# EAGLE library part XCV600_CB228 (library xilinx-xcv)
xcv600_cb228 edit this description Auto generated by make-symbol-device-package-bsdl.ulp Rev. 26 Source: xcv600_cb228.bsd
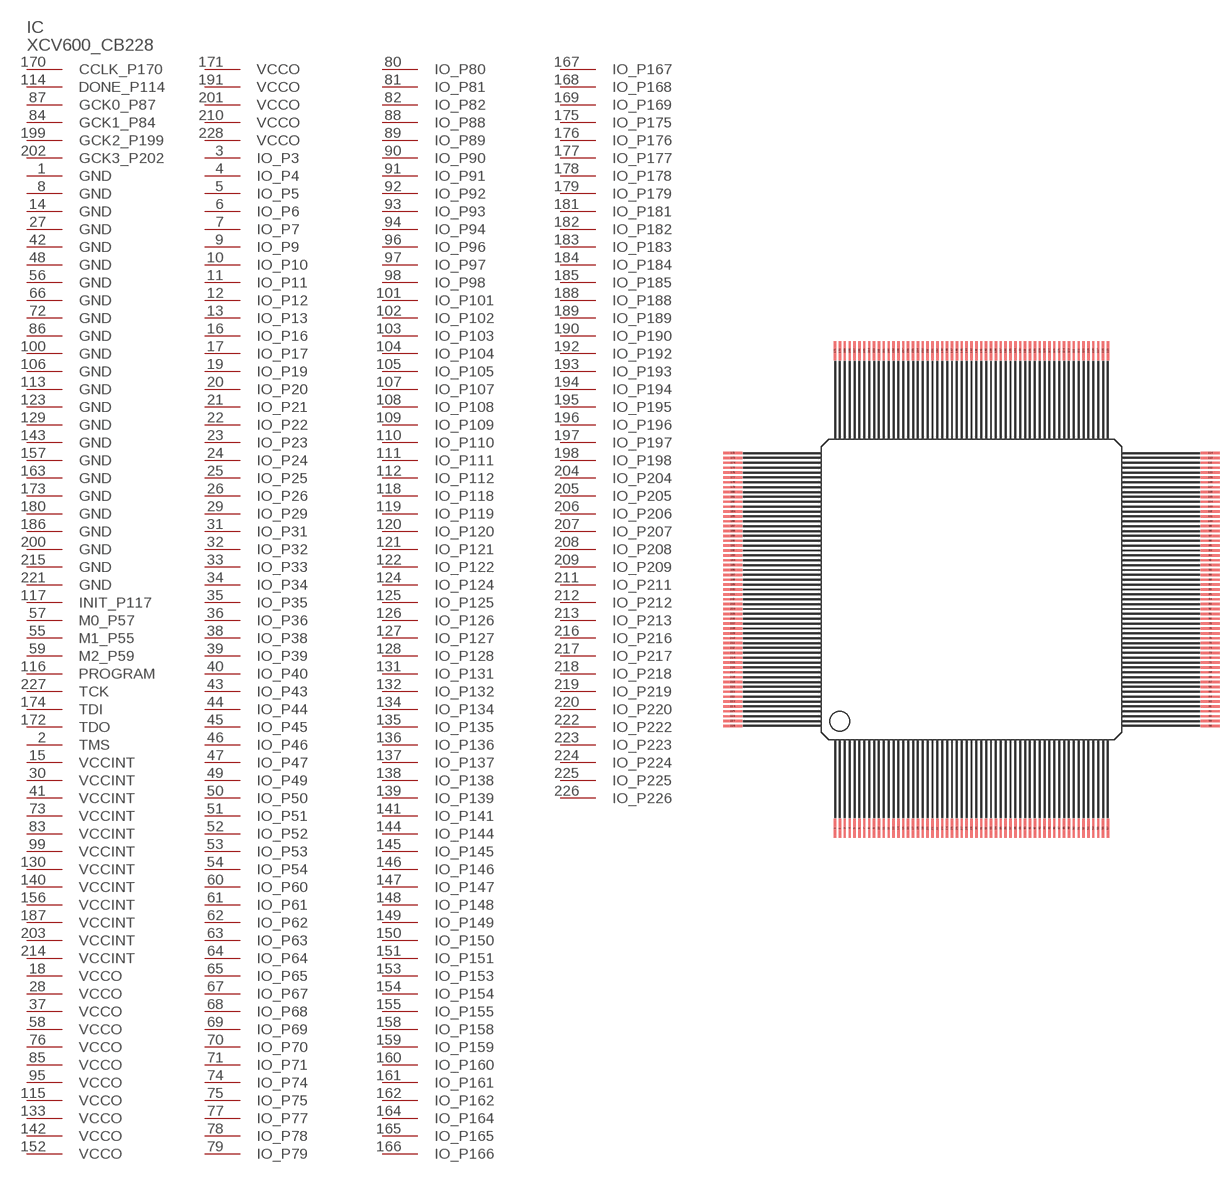
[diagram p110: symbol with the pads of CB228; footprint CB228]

Designator prefix IC

## XCV600_CB228 (OC_FARNELL: unknown; OC_NEWARK: unknown)  [CB228]
1  GND  pwr
2  TMS  in
3  IO_P3
4  IO_P4
5  IO_P5
6  IO_P6
7  IO_P7
8  GND  pwr
9  IO_P9
10  IO_P10
11  IO_P11
12  IO_P12
13  IO_P13
14  GND  pwr
15  VCCINT  pwr
16  IO_P16
17  IO_P17
18  VCCO  pwr
19  IO_P19
20  IO_P20
21  IO_P21
22  IO_P22
23  IO_P23
24  IO_P24
25  IO_P25
26  IO_P26
27  GND  pwr
28  VCCO  pwr
29  IO_P29
30  VCCINT  pwr
31  IO_P31
32  IO_P32
33  IO_P33
34  IO_P34
35  IO_P35
36  IO_P36
37  VCCO  pwr
38  IO_P38
39  IO_P39
40  IO_P40
41  VCCINT  pwr
42  GND  pwr
43  IO_P43
44  IO_P44
45  IO_P45
46  IO_P46
47  IO_P47
48  GND  pwr
49  IO_P49
50  IO_P50
51  IO_P51
52  IO_P52
53  IO_P53
54  IO_P54
55  M1_P55  in
56  GND  pwr
57  M0_P57  in
58  VCCO  pwr
59  M2_P59  in
60  IO_P60
61  IO_P61
62  IO_P62
63  IO_P63
64  IO_P64
65  IO_P65
66  GND  pwr
67  IO_P67
68  IO_P68
69  IO_P69
70  IO_P70
71  IO_P71
72  GND  pwr
73  VCCINT  pwr
74  IO_P74
75  IO_P75
76  VCCO  pwr
77  IO_P77
78  IO_P78
79  IO_P79
80  IO_P80
81  IO_P81
82  IO_P82
83  VCCINT  pwr
84  GCK1_P84  in
85  VCCO  pwr
86  GND  pwr
87  GCK0_P87  in
88  IO_P88
89  IO_P89
90  IO_P90
91  IO_P91
92  IO_P92
93  IO_P93
94  IO_P94
95  VCCO  pwr
96  IO_P96
97  IO_P97
98  IO_P98
99  VCCINT  pwr
100  GND  pwr
101  IO_P101
102  IO_P102
103  IO_P103
104  IO_P104
105  IO_P105
106  GND  pwr
107  IO_P107
108  IO_P108
109  IO_P109
110  IO_P110
111  IO_P111
112  IO_P112
113  GND  pwr
114  DONE_P114
115  VCCO  pwr
116  PROGRAM  in
117  INIT_P117
118  IO_P118
119  IO_P119
120  IO_P120
121  IO_P121
122  IO_P122
123  GND  pwr
124  IO_P124
125  IO_P125
126  IO_P126
127  IO_P127
128  IO_P128
129  GND  pwr
130  VCCINT  pwr
131  IO_P131
132  IO_P132
133  VCCO  pwr
134  IO_P134
135  IO_P135
136  IO_P136
137  IO_P137
138  IO_P138
139  IO_P139
140  VCCINT  pwr
141  IO_P141
142  VCCO  pwr
143  GND  pwr
144  IO_P144
145  IO_P145
146  IO_P146
147  IO_P147
148  IO_P148
149  IO_P149
150  IO_P150
151  IO_P151
152  VCCO  pwr
153  IO_P153
154  IO_P154
155  IO_P155
156  VCCINT  pwr
157  GND  pwr
158  IO_P158
159  IO_P159
160  IO_P160
161  IO_P161
162  IO_P162
163  GND  pwr
164  IO_P164
165  IO_P165
166  IO_P166
167  IO_P167
168  IO_P168
169  IO_P169
170  CCLK_P170
171  VCCO  pwr
172  TDO  out
173  GND  pwr
174  TDI  in
175  IO_P175
176  IO_P176
177  IO_P177
178  IO_P178
179  IO_P179
180  GND  pwr
181  IO_P181
182  IO_P182
183  IO_P183
184  IO_P184
185  IO_P185
186  GND  pwr
187  VCCINT  pwr
188  IO_P188
189  IO_P189
190  IO_P190
191  VCCO  pwr
192  IO_P192
193  IO_P193
194  IO_P194
195  IO_P195
196  IO_P196
197  IO_P197
198  IO_P198
199  GCK2_P199  in
200  GND  pwr
201  VCCO  pwr
202  GCK3_P202  in
203  VCCINT  pwr
204  IO_P204
205  IO_P205
206  IO_P206
207  IO_P207
208  IO_P208
209  IO_P209
210  VCCO  pwr
211  IO_P211
212  IO_P212
213  IO_P213
214  VCCINT  pwr
215  GND  pwr
216  IO_P216
217  IO_P217
218  IO_P218
219  IO_P219
220  IO_P220
221  GND  pwr
222  IO_P222
223  IO_P223
224  IO_P224
225  IO_P225
226  IO_P226
227  TCK  in
228  VCCO  pwr

## Footprint CB228 (pad centres in mm)
Ceramic Brazed CQFP (CB228) Package Source: cb228.pdf
smd 0.305 x 2.54: 1 -17.78,-31.115; 2 -17.145,-31.115; 3 -16.51,-31.115; 4 -15.875,-31.115; 5 -15.24,-31.115; 6 -14.605,-31.115; 7 -13.97,-31.115; 8 -13.335,-31.115; 9 -12.7,-31.115; 10 -12.065,-31.115; 11 -11.43,-31.115; 12 -10.795,-31.115; 13 -10.16,-31.115; 14 -9.525,-31.115; 15 -8.89,-31.115; 16 -8.255,-31.115; 17 -7.62,-31.115; 18 -6.985,-31.115; 19 -6.35,-31.115; 20 -5.715,-31.115; 21 -5.08,-31.115; 22 -4.445,-31.115; 23 -3.81,-31.115; 24 -3.175,-31.115; 25 -2.54,-31.115; 26 -1.905,-31.115; 27 -1.27,-31.115; 28 -0.635,-31.115; 29 0,-31.115; 30 0.635,-31.115; 31 1.27,-31.115; 32 1.905,-31.115; 33 2.54,-31.115; 34 3.175,-31.115; 35 3.81,-31.115; 36 4.445,-31.115; 37 5.08,-31.115; 38 5.715,-31.115; 39 6.35,-31.115; 40 6.985,-31.115; 41 7.62,-31.115; 42 8.255,-31.115; 43 8.89,-31.115; 44 9.525,-31.115; 45 10.16,-31.115; 46 10.795,-31.115; 47 11.43,-31.115; 48 12.065,-31.115; 49 12.7,-31.115; 50 13.335,-31.115; 51 13.97,-31.115; 52 14.605,-31.115; 53 15.24,-31.115; 54 15.875,-31.115; 55 16.51,-31.115; 56 17.145,-31.115; 57 17.78,-31.115; 115 17.78,31.115; 116 17.145,31.115; 117 16.51,31.115; 118 15.875,31.115; 119 15.24,31.115; 120 14.605,31.115; 121 13.97,31.115; 122 13.335,31.115; 123 12.7,31.115; 124 12.065,31.115; 125 11.43,31.115; 126 10.795,31.115; 127 10.16,31.115; 128 9.525,31.115; 129 8.89,31.115; 130 8.255,31.115; 131 7.62,31.115; 132 6.985,31.115; 133 6.35,31.115; 134 5.715,31.115; 135 5.08,31.115; 136 4.445,31.115; 137 3.81,31.115; 138 3.175,31.115; 139 2.54,31.115; 140 1.905,31.115; 141 1.27,31.115; 142 0.635,31.115; 143 0,31.115; 144 -0.635,31.115; 145 -1.27,31.115; 146 -1.905,31.115; 147 -2.54,31.115; 148 -3.175,31.115; 149 -3.81,31.115; 150 -4.445,31.115; 151 -5.08,31.115; 152 -5.715,31.115; 153 -6.35,31.115; 154 -6.985,31.115; 155 -7.62,31.115; 156 -8.255,31.115; 157 -8.89,31.115; 158 -9.525,31.115; 159 -10.16,31.115; 160 -10.795,31.115; 161 -11.43,31.115; 162 -12.065,31.115; 163 -12.7,31.115; 164 -13.335,31.115; 165 -13.97,31.115; 166 -14.605,31.115; 167 -15.24,31.115; 168 -15.875,31.115; 169 -16.51,31.115; 170 -17.145,31.115; 171 -17.78,31.115
smd 2.54 x 0.305: 58 31.115,-17.78; 59 31.115,-17.145; 60 31.115,-16.51; 61 31.115,-15.875; 62 31.115,-15.24; 63 31.115,-14.605; 64 31.115,-13.97; 65 31.115,-13.335; 66 31.115,-12.7; 67 31.115,-12.065; 68 31.115,-11.43; 69 31.115,-10.795; 70 31.115,-10.16; 71 31.115,-9.525; 72 31.115,-8.89; 73 31.115,-8.255; 74 31.115,-7.62; 75 31.115,-6.985; 76 31.115,-6.35; 77 31.115,-5.715; 78 31.115,-5.08; 79 31.115,-4.445; 80 31.115,-3.81; 81 31.115,-3.175; 82 31.115,-2.54; 83 31.115,-1.905; 84 31.115,-1.27; 85 31.115,-0.635; 86 31.115,0; 87 31.115,0.635; 88 31.115,1.27; 89 31.115,1.905; 90 31.115,2.54; 91 31.115,3.175; 92 31.115,3.81; 93 31.115,4.445; 94 31.115,5.08; 95 31.115,5.715; 96 31.115,6.35; 97 31.115,6.985; 98 31.115,7.62; 99 31.115,8.255; 100 31.115,8.89; 101 31.115,9.525; 102 31.115,10.16; 103 31.115,10.795; 104 31.115,11.43; 105 31.115,12.065; 106 31.115,12.7; 107 31.115,13.335; 108 31.115,13.97; 109 31.115,14.605; 110 31.115,15.24; 111 31.115,15.875; 112 31.115,16.51; 113 31.115,17.145; 114 31.115,17.78; 172 -31.115,17.78; 173 -31.115,17.145; 174 -31.115,16.51; 175 -31.115,15.875; 176 -31.115,15.24; 177 -31.115,14.605; 178 -31.115,13.97; 179 -31.115,13.335; 180 -31.115,12.7; 181 -31.115,12.065; 182 -31.115,11.43; 183 -31.115,10.795; 184 -31.115,10.16; 185 -31.115,9.525; 186 -31.115,8.89; 187 -31.115,8.255; 188 -31.115,7.62; 189 -31.115,6.985; 190 -31.115,6.35; 191 -31.115,5.715; 192 -31.115,5.08; 193 -31.115,4.445; 194 -31.115,3.81; 195 -31.115,3.175; 196 -31.115,2.54; 197 -31.115,1.905; 198 -31.115,1.27; 199 -31.115,0.635; 200 -31.115,0; 201 -31.115,-0.635; 202 -31.115,-1.27; 203 -31.115,-1.905; 204 -31.115,-2.54; 205 -31.115,-3.175; 206 -31.115,-3.81; 207 -31.115,-4.445; 208 -31.115,-5.08; 209 -31.115,-5.715; 210 -31.115,-6.35; 211 -31.115,-6.985; 212 -31.115,-7.62; 213 -31.115,-8.255; 214 -31.115,-8.89; 215 -31.115,-9.525; 216 -31.115,-10.16; 217 -31.115,-10.795; 218 -31.115,-11.43; 219 -31.115,-12.065; 220 -31.115,-12.7; 221 -31.115,-13.335; 222 -31.115,-13.97; 223 -31.115,-14.605; 224 -31.115,-15.24; 225 -31.115,-15.875; 226 -31.115,-16.51; 227 -31.115,-17.145; 228 -31.115,-17.78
